PROGRAM MAIN
VAR
	fbEventlogger : FB_TcEventLogger;
	fbAlarm: FB_TcAlarm;
	fbMessage: FB_TcMessage;
	
	bAlarm: BOOL;
	bMessage : BOOL;
	bIsInitalized: BOOL;
	bClearAlarm: BOOL;
	bConfirmAlarm: BOOL;
END_VAR

IF NOT bIsInitalized THEN
	bIsInitalized := TRUE;
	fbMessage.CreateEx(TC_Events.MyEvents.Start, 0);
	fbAlarm.CreateEx(TC_Events.MyEvents.Stop, TRUE, 0);
END_IF

IF bMessage THEN
	bMessage := FALSE;
	fbMessage.Send(0);
END_IF

IF bAlarm THEN
	bAlarm := FALSE;
	fbAlarm.Raise(0);
END_IF

IF bClearAlarm THEN
	bClearAlarm := FALSE;
	fbAlarm.Clear(0, FALSE);
END_IF

END_PROGRAM
